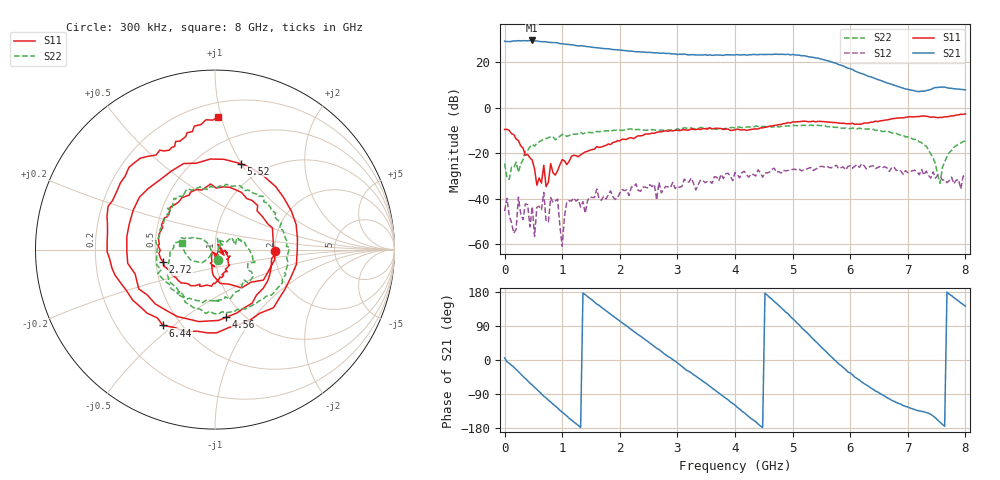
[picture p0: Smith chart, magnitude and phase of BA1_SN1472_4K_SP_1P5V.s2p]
! VC=1.5V IC=6.89mA
# HZ S DB R 50.00
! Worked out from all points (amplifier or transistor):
!   201 points, 300 kHz to 8 GHz, reference 50 ohm
!   highest |S21| = 29.7 dB at 480.3 MHz (marker M1)
!   |S21| within 3 dB of that: start of sweep to 1.518 GHz
!   unconditionally stable (mu >= 1): start of sweep to 3.754 GHz; 3.765 GHz to 3.828 GHz; 5.898 GHz to end of sweep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
!   at 1.32 GHz: K = 2.99, MAG = 27.8 dB, |S12| = -43.6 dB
!   at 4 GHz: K = 0.90, MSG = 25.8 dB, |S12| = -28.4 dB
!   at 8 GHz: K = 2.53, MAG = 11.8 dB, |S12| = -29.3 dB
!   S11 on the Smith chart (normalised r, x): 300 kHz: 2.01, -0.03; 2.72 GHz: 0.55, -0.08; 4.56 GHz: 0.84, -0.74; 5.52 GHz: 0.78, +0.99; 6.44 GHz: 0.40, -0.46; 8 GHz: 0.30, +0.98
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300000  -9.49 -1.0  29.35 5.7  -45.37 -24.1  -24.53 -71.7
2.40291e8  -14.39 -81.3  29.60 -31.0  -39.26 95.5  -28.27 63.0
4.80282e8  -23.00 -103.8  29.69 -65.8  -43.50 31.2  -16.02 16.0
6.802745e8  -25.21 -85.4  29.18 -95.6  -37.23 21.6  -13.64 -9.2
9.202655e8  -27.62 -21.8  28.65 -126.6  -40.13 84.4  -13.39 -31.9
1.360249e9  -19.98 -43.2  27.28 176.6  -41.26 19.8  -11.42 -77.7
1.60024e9  -17.02 -61.2  26.55 147.8  -35.71 -11.7  -10.34 -103.3
1.960226e9  -14.45 -90.1  25.58 107.8  -39.70 -28.4  -9.69 -138.5
2.320213e9  -12.29 -124.2  24.72 66.7  -36.29 -63.8  -9.47 -166.2
2.6802e9  -10.54 -161.3  24.15 27.7  -32.72 -78.6  -9.90 161.8
2.720198e9  -10.54 -166.8  24.02 22.9  -37.41 -94.6  -9.73 160.5
3.120183e9  -9.57 147.8  23.73 -22.3  -31.33 -144.4  -8.73 128.6
3.48017e9  -9.12 106.9  23.46 -59.8  -32.91 -153.3  -9.01 111.3
4.00015e9  -9.69 25.6  23.25 -118.9  -28.44 167.7  -8.76 75.2
4.560129e9  -8.36 -80.5  23.52 171.2  -28.64 114.7  -8.31 35.9
5.000112e9  -6.16 -171.0  23.55 109.2  -27.07 79.3  -7.68 2.0
5.360099e9  -5.84 110.0  22.23 55.1  -27.56 44.8  -7.78 -23.3
5.520093e9  -6.02 73.4  21.35 30.6  -25.76 27.2  -7.79 -34.3
5.960076e9  -6.97 -29.5  17.48 -31.5  -25.79 -14.1  -8.94 -79.5
6.440058e9  -5.80 -124.5  12.87 -82.1  -26.74 -69.9  -9.91 -122.8
6.68005e9  -5.09 -160.3  10.70 -102.5  -28.00 -96.9  -10.51 -152.3
8e9  -2.63 88.5  7.96 141.9  -29.30 176.9  -14.57 168.7
